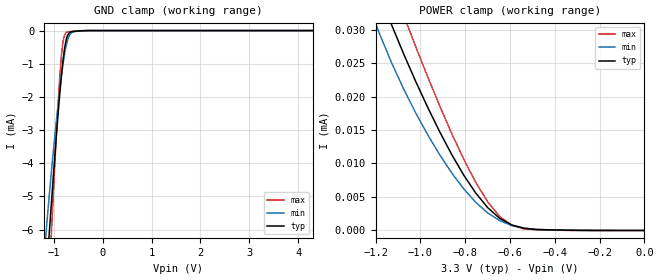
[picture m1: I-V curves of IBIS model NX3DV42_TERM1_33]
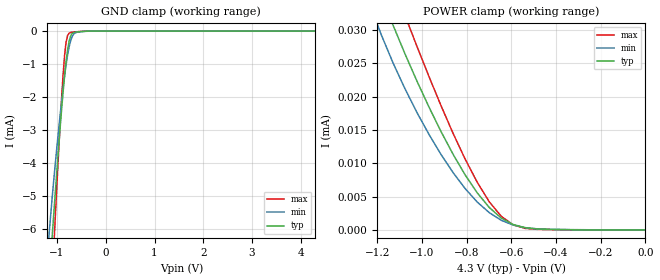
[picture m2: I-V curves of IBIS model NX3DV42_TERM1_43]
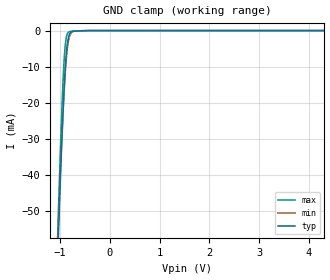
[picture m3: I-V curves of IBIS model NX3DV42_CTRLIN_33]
| NXP Semiconductors
| Logic Products Group
| IBIS model of NX3DV42GU
| DUAL HIGH-SPEED USB 2.0 DPDT ANALOG SWITCH
|[Packages]:
|[Package1]: XQFN10 (GU) 10-pins Package
[IBIS Ver]   3.2
[File Name]   nx3dv42gu.ibs
[File Rev]   1.0
[Date]   27-Jul-2012
[Source]   File created from simulations by LPG
   NXP Semiconductors Nijmegen
[Notes]   V1.0   Ibis model.
   Revision History
   Version Date   Author/ Description
   Editor
   1.0   July 2012   RRV   Initial Model
   Remarks: - The Power Clamp curves have been omitted from the input
   since the is no power clamp diode.
   - IBISCHK 5.0.3 used
   - Following notes/warnings are caused by normal switch behaviour:
   'Series_MOSFET has Decreasing Current'
   'Series_MOSFET data is non-monotonic'
[Disclaimer]
   NXP Semiconductors warrants and represents that the IBIS model
   identified herein is owned by NXP Semiconductors (NXP). The
   model provided is not warranted as fully representing all of the
   operating characteristics and specifications of the semiconductor
   products to which the model relates.  Moreover, unless there is a
   signed, written agreement to the contrary, this IBIS model is
   furnished on an "as is" basis without support or warranty of any
   kind, either expressed or implied, regarding the use thereof, and
   NXP specifically disclaims all implied warranties of
   merchantability and fitness of the model for any purpose.
   NXP does not assume any liability arising out of the application
   or use of this IBIS model including infringement of patents and
   copyrights, nor does NXP convey any license under its patents and
   copyrights or the rights of others.
   NXP provides IBIS models as a service to our customers. You and
   your company shall not distribute, convey, sell, or give these models
   to anyone else without receiving prior written permission from
   NXP.
   NXP reserves the right to make changes without notice to these
   IBIS models to improve reliability, function, or design.
   Please be aware that your receipt and subsequent use of the IBIS
   information provided shall serve as acceptance of the terms and
   conditions of this agreement.  If you do not accept these terms,
   you should return or destroy the IBIS models and any other
   accompanying information immediately.
[Copyright]
   (C) Copyright 2012 NXP Semiconductors
   All rights reserved
|   Info for  XQFN10 (GU) 10-pins Package
[Component]   NX3DV42_GU
[Manufacturer]   NXP Semiconductors
[Package]
|   Typ   Min   Max
R_pkg   3.587E-02   3.369E-02   3.832E-02
L_pkg   4.581E-10   4.300E-10   4.894E-10
C_pkg   1.292E-13   1.164E-13   1.473E-13
[Pin] signal_name   model_name   R_pin   L_pin   C_pin
   1   DP   NX3DV42_TERM1 3.526E-02 4.502E-10 1.181E-13
   2   DM   NX3DV42_TERM1 3.385E-02 4.322E-10 1.164E-13
   3   GND   GND 3.798E-02 4.851E-10 1.473E-13
   4   HSD1M   NX3DV42_TERM1 3.369E-02 4.300E-10 1.421E-13
   5   HSD1P   NX3DV42_TERM1 3.832E-02 4.894E-10 1.216E-13
   6   HSD2M   NX3DV42_TERM1 3.385E-02 4.322E-10 1.164E-13
   7   HSD2P   NX3DV42_TERM1 3.527E-02 4.503E-10 1.440E-13
   8   OEN   NX3DV42_CTRLIN 3.802E-02 4.856E-10 1.473E-13
   9   VCC   POWER 3.448E-02 4.403E-10 1.172E-13
   10   S   NX3DV42_CTRLIN 3.803E-02 4.857E-10 1.213E-13
[Series Pin Mapping]  pin_2  model_name   function_table_group
1   4   NX3DV42_SWITCH1   1
1   6   NX3DV42_SWITCH1   2
4   1   NX3DV42_SWITCH1   3
6   1   NX3DV42_SWITCH1   4
2   5   NX3DV42_SWITCH1   1
2   7   NX3DV42_SWITCH1   2
5   2   NX3DV42_SWITCH1   3
7   2   NX3DV42_SWITCH1   4
[Series Switch Groups]
| Function Group States
On 1 /   | D+/D- to HSD1+/HSD1-, S=Low,  En=Low
On 2 /   | D+/D- to HSD2+/HSD2-, S=High, En=Low
On 3 /   | HSD1+/HSD1- to D+/D-, S=Low,  En=Low
On 4 /   | HSD2+/HSD2- to D+/D-, S=High, En=Low
Off 1 2 3 4 /   | En=High
[Model Selector]   NX3DV42_SWITCH1
NX3DV42_SWITCH1_33   3.3V-Vcc Series switch model
NX3DV42_SWITCH1_43   4.3V-Vcc Series switch model
[Model Selector]   NX3DV42_TERM1
NX3DV42_TERM1_33   3.3V-Vcc Series Switch I/O model
NX3DV42_TERM1_43   4.3V-Vcc Series Switch I/O model
[Model Selector]   NX3DV42_CTRLIN
NX3DV42_CTRLIN_33   3.3V-Vcc input model
NX3DV42_CTRLIN_43   4.3V-Vcc input model
|   Model NX3DV42_SWITCH1_33
[Model]   NX3DV42_SWITCH1_33
Model_type   Series_switch
C_comp   7.223pF   6.798pF   7.526pF
| ON capacitance of switch
|Ambient temperature:   25   85   -40
[Temperature Range]   30   90   -35
[Voltage Range]   3.3   3.0   3.6
[Off]
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[On]
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|   Model NX3DV42_SWITCH1_43
[Model]   NX3DV42_SWITCH1_43
Model_type   Series_switch
C_comp   7.223pF   6.798pF   7.526pF
| ON capacitance of switch
|Ambient temperature:   25   85   -40
[Temperature Range]   30   90   -35
[Voltage Range]   4.3   4.3   4.3
[Off]
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[On]
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| Models and submodels in the file (6): NX3DV42_TERM1_33 (Terminator), NX3DV42_SWITCH1_33 (Series_switch), NX3DV42_TERM1_43 (Terminator), NX3DV42_SWITCH1_43 (Series_switch), NX3DV42_CTRLIN_33 (Input), NX3DV42_CTRLIN_43 (Input)
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| Remark: If your software does not support the Model Selector
|   Please comment out the lines of the Model Selector, which
|   contain the name of the Model, except the one you want to use.
|   Model NX3DV42_TERM1_33
[Model]   NX3DV42_TERM1_33
Model_type   Terminator
C_comp   7.223pF   6.798pF   7.526pF
| ON capacitance of switch
|Ambient temperature:   25   85   -40
[Temperature Range]   30   90   -35
[Voltage Range]   3.3   3.0   3.6
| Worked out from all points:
|   GND clamp passes 1 mA (typ) near -0.82 V on its own axis
|   POWER clamp passes 1 mA (typ) near -2.67 V on its own axis
|Process Range   nominal   slow   fast
[GND_clamp]
|   voltage   I(typ)   I(min)   I(max)
-4.3V     -2.17A     -1.847A    -2.547A
-1.156V   -7.48mA    -6.066mA   -9.367mA
-1.094V   -6.137mA   -4.981mA   -7.446mA
-1.062V   -5.482mA   -4.469mA   -6.496mA
-1.031V   -4.837mA   -3.975mA   -5.558mA
-906.2mV  -2.404mA   -2.15mA    -2.064mA
-843.8mV  -1.356mA   -1.361mA   -740.6uA
-812.5mV  -915.8uA   -1.017mA   -332.5uA
-750mV    -299uA     -474.7uA   -62.81uA
-656.2mV  -44.73uA   -91.84uA   -27.59uA
-406.2mV  -4.726uA   -7.593uA   -1.957uA
4.3V      0A         0A         0A
[POWER_clamp]
|   voltage   I(typ)   I(min)   I(max)
-4.3V     3.367mA    2.572mA    4.722mA
-1.236V   40.39uA    34.19uA    46.96uA
-1.183V   35.35uA    29.36uA    41.88uA
-1.129V   30.72uA    25.05uA    36.95uA
-1.075V   26.38uA    21.15uA    32.16uA
-1.021V   22.28uA    17.58uA    27.48uA
-913.7mV  14.73uA    11.3uA     18.6uA
-806.3mV  8.25uA     6.205uA    10.62uA
-698.7mV  3.384uA    2.603uA    4.238uA
-645mV    1.786uA    1.455uA    2.054uA
-537.5mV  334.4nA    347.5nA    232.6nA
0V        64.42pA    71.44pA    73.44pA
|   Model NX3DV42_TERM1_43
[Model]   NX3DV42_TERM1_43
Model_type   Terminator
C_comp   7.073pF   6.794pF   7.367pF
| ON capacitance of switch
|Ambient temperature:   25   85   -40
[Temperature Range]   30   90   -35
[Voltage Range]   4.3   4.3   4.3
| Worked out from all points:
|   GND clamp passes 1 mA (typ) near -0.82 V on its own axis
|   POWER clamp passes 1 mA (typ) near -2.67 V on its own axis
|Process Range   nominal   slow   fast
[GND_clamp]
|   voltage   I(typ)   I(min)   I(max)
-4.3V     -2.17A     -1.847A    -2.547A
-1.156V   -7.48mA    -6.066mA   -9.367mA
-1.094V   -6.137mA   -4.981mA   -7.446mA
-1.062V   -5.482mA   -4.469mA   -6.496mA
-1.031V   -4.837mA   -3.975mA   -5.558mA
-906.2mV  -2.404mA   -2.15mA    -2.064mA
-843.8mV  -1.356mA   -1.361mA   -740.6uA
-812.5mV  -915.8uA   -1.017mA   -332.5uA
-750mV    -299uA     -474.7uA   -62.81uA
-656.2mV  -44.73uA   -91.84uA   -27.59uA
-406.2mV  -4.726uA   -7.593uA   -1.957uA
4.3V      0A         0A         0A
[POWER_clamp]
|   voltage   I(typ)   I(min)   I(max)
-4.3V     3.367mA    2.572mA    4.722mA
-1.236V   40.39uA    34.19uA    46.96uA
-1.183V   35.35uA    29.36uA    41.88uA
-1.129V   30.72uA    25.05uA    36.95uA
-1.075V   26.38uA    21.15uA    32.16uA
-1.021V   22.28uA    17.58uA    27.48uA
-913.7mV  14.73uA    11.3uA     18.6uA
-806.3mV  8.25uA     6.205uA    10.62uA
-698.7mV  3.384uA    2.603uA    4.238uA
-645mV    1.786uA    1.455uA    2.054uA
-537.5mV  334.4nA    347.5nA    232.6nA
0V        64.42pA    71.44pA    73.44pA
|   Model NX3DV42_CTRLIN_33
[Model]   NX3DV42_CTRLIN_33
Model_type   Input
Vinl = 0.5V
Vinh = 1.3V
C_comp   0.867pF   0.821pF   0.937pF
[Model Spec]
| Note: The input and output voltage ratings may be exceeded if the input and
|   output current ratings are observed (please refer to the data sheet)
|   Subparameter   typ   min   max
| Thresholds
Vinl   0.5   0.5   0.5
Vinh   1.3   1.3   1.3
| Overshoot
S_overshoot_high   3.6   3.6   3.6
S_overshoot_low   -0.5   -0.5   -0.5
D_overshoot_high   5.5   5.5   5.5
D_overshoot_low   -0.95   -0.9   -1.0
D_overshoot_time   3n   3n   3n
|Ambient temperature:   25   85   -40
[Temperature Range]   30   90   -35
[Voltage Range]   3.3   3.0   3.6
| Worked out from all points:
|   GND clamp passes 1 mA (typ) near -0.81 V on its own axis
|Process Range   nominal   slow   fast
[GND_clamp]
|   voltage   I(typ)   I(min)   I(max)
-4.3V     -1.553A    -1.422A    -1.69A
-1.062V   -67.87mA   -63.41mA   -61.74mA
-1.047V   -61.37mA   -57.56mA   -54.65mA
-1.031V   -55mA      -51.83mA   -47.72mA
-968.8mV  -31.2mA    -30.51mA   -22.4mA
-921.9mV  -16.31mA   -17.15mA   -8.299mA
-875mV    -6.075mA   -7.52mA    -1.726mA
-843.8mV  -2.534mA   -3.684mA   -580.6uA
-812.5mV  -990.4uA   -1.642mA   -277.3uA
-734.4mV  -207.8uA   -256.9uA   -137.5uA
-437.5mV  -7.087uA   -16.06uA   -2.371uA
4.3V      0A         0A         0A
